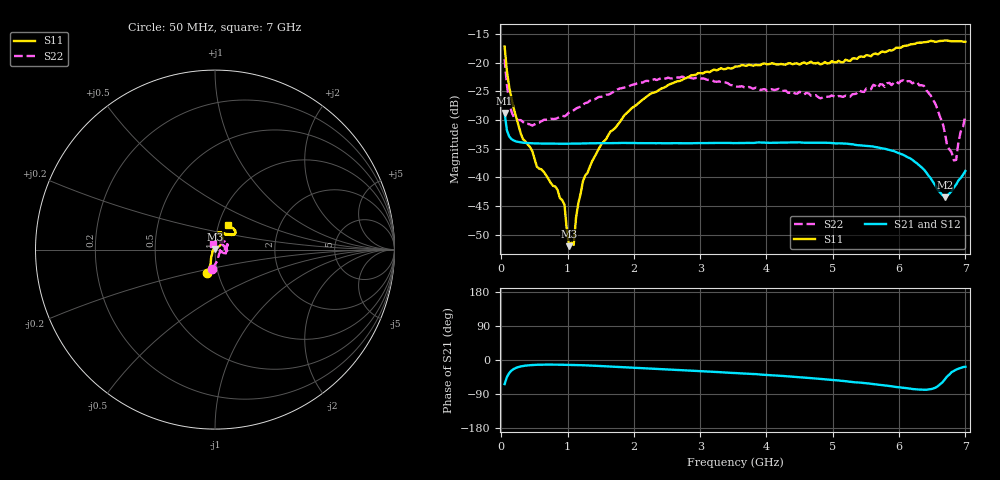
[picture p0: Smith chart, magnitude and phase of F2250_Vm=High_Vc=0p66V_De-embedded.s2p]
! Integrated Device Technology
! Corporate Headquarters
! 6024 Silver Creek Valley Road
! San Jose, CA 95138  USA
! Phone:  1-408-284-8200
! Toll Free:  1-800-223-1366
! Webpage:  http://www.idt.com/
! Timing and RF Division
! 515 Groton Road, Suite 102
! Westford, MA 01886-6024
! Device:  F2250
! Description: Voltage Variable RF Attenuator
! Frequency:  50.0 -  6000.00 MHz
! Package:  3x3 mm Thin QFN Plastic Package: 16 pin
! Ports:  2 RF, 3 DC
!  Pin  1  = GND
!  Pin  2  = NC
!  Pin  3  = RF1  = Port 1
!  Pin  4  = NC
!  Pin  5  = GND
!  Pin  6  = GND
!  Pin  7  = GND
!  Pin  8  = GND
!  Pin  9  = NC
!  Pin 10  = RF2  = Port 2
!  Pin 11  = NC
!  Pin 12  = GND
!  Pin 13  = GND
!  Pin 14  = VCNTRL
!  Pin 15  = VDD
!  Pin 16  = VMODE
! Vcntrl:  0.660 Volts
! Vmode:  +3.300 Volts
! Vdd:  +3.30  Volts
! Current:  1.284 mA
! Data:  The device was measured on a the F2250 evaluation board which has
!  individual transmission lines to the RF pins.  Data was collected
!  using a calibrated network analyzer.  The evaluation board was
!  de-embedded using a TRL calibration technique.
!  The reference plane is the edge of the package pin.
! Misc:  SN 10
!  Action Tracker AT0258
! Date Measured:  2014-11-26
! Date:  2015-10-15  MJV
! Note:
!  Integrated Device Technology supplies this data as a sample of measured
!  data at the package pin for this product.  Your particular data for this
!  product may vary.
!  Data was taken at 25 degrees C.
!  Integrated Device Technology reserves the right to change this data at anytime.
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# GHz S dB R 50
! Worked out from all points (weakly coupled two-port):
!   201 points, 50 MHz to 7 GHz, reference 50 ohm
!   highest |S21| = -28.75 dB at 50 MHz (marker M1); lowest = -43.4 dB at 6.687 GHz (marker M2)
!   lowest |S11| = -52.0 dB at 1.023 GHz (marker M3), VSWR 1.01, Z = 49.8 + j0.169 ohm
!   |S11| at or under -10 dB: start of sweep to end of sweep
!   |S22| runs from -37.0 to -19.3 dB; largest |S21 - S12| = 4.8e-05
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0.05  -17.16 -108.2  -28.75 -63.5  -28.75 -63.5  -19.35 -98.0
0.1195  -24.20 -111.5  -32.85 -34.4  -32.85 -34.4  -26.81 -67.1
0.22375  -29.46 -121.9  -33.72 -20.7  -33.72 -20.7  -29.91 -42.8
0.5365  -38.11 -153.6  -34.06 -12.7  -34.06 -12.7  -30.54 -9.5
0.9535  -44.77 171.2  -34.12 -12.6  -34.12 -12.6  -29.36 -1.1
1.023  -51.97 137.7  -34.10 -12.8  -34.11 -12.8  -28.66 0.3
1.0925  -51.75 82.1  -34.10 -13.1  -34.10 -13.1  -28.27 1.6
1.12725  -47.01 56.2  -34.09 -13.3  -34.09 -13.3  -27.99 1.1
1.2315  -40.67 38.5  -34.06 -13.8  -34.06 -13.8  -27.30 0.6
1.6485  -31.98 40.3  -34.01 -17.0  -34.02 -17.1  -25.39 8.1
2.37825  -24.75 46.3  -34.01 -23.6  -34.01 -23.7  -22.85 18.2
3.525  -20.67 71.5  -34.00 -34.3  -33.99 -34.4  -24.00 45.8
4.7065  -20.09 71.9  -33.91 -48.3  -33.92 -48.3  -25.68 51.6
5.2625  -19.69 53.1  -34.16 -57.4  -34.16 -57.4  -25.89 26.2
5.85325  -17.81 40.4  -35.21 -68.6  -35.21 -68.7  -23.49 -1.3
6.3745  -16.41 40.8  -38.61 -78.5  -38.62 -78.6  -24.01 -18.2
6.54825  -16.35 44.6  -41.42 -73.0  -41.44 -73.0  -27.17 -21.4
6.68725  -16.13 47.7  -43.44 -51.6  -43.45 -51.4  -32.03 -3.6
6.722  -16.11 49.2  -43.22 -44.0  -43.19 -43.9  -34.28 1.5
6.861  -16.23 54.4  -41.22 -25.3  -41.20 -25.4  -36.92 66.4
6.89575  -16.23 56.4  -40.50 -23.0  -40.47 -23.0  -33.74 80.5
7  -16.35 62.3  -38.86 -17.8  -38.82 -17.9  -29.23 109.4
